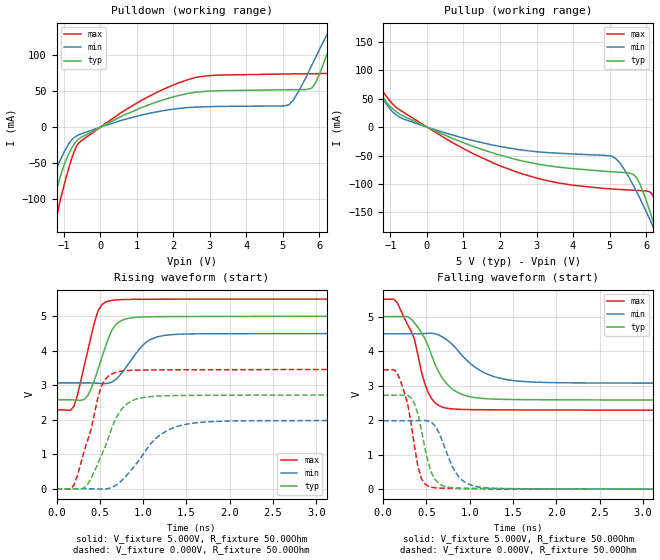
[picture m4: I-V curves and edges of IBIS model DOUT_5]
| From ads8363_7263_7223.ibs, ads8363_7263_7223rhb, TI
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|   Output 5.0V Model
[Model]   DOUT_5
Model_type   Output
|Signals   SDOA, SDOB
Vmeas = 2.413V
Cref = 30.00pF
| C_comp   obtained at 36MHz
| variable   typ   min   max
|C_comp Output Low
C_comp   3.625pF   2.838pF   4.470pF
|C_comp Output High
|C_comp   3.802pF   3.032pF   4.673pF
[Model Spec]
Vmeas   2.41V   2.19V   2.78V
Vref   2.50V   0.50V   3.00V
|Junction Temperature
[Temperature Range]   40.0   125.0   -40.0
[Voltage range]   5.0V   4.50V   5.50V
[pullup reference]   5.0V   4.50V   5.50V
[power clamp reference]   5.0V   4.50V   5.50V
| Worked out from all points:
|   slope of the pulldown table from 0 to 0.75 V, typ, clamps not added: 39.7 ohm
|   slope of the pullup table from 0 to 0.75 V, typ, clamps not added: 35.6 ohm
|   falling waveform, V_fixture 5.000V, R_fixture 50.00Ohm: 20-80 % time 285ps typ, 394ps min, 237ps max; typ from 5 V to 2.58 V
|   rising waveform, V_fixture 5.000V, R_fixture 50.00Ohm: 20-80 % time 201ps typ, 268ps min, 180ps max; typ from 2.58 V to 5 V
|   rising waveform, V_fixture 0.000V, R_fixture 50.00Ohm: 20-80 % time 270ps typ, 399ps min, 217ps max; typ from 0 V to 2.72 V
|   falling waveform, V_fixture 0.000V, R_fixture 50.00Ohm: 20-80 % time 148ps typ, 211ps min, 150ps max; typ from 2.72 V to 0 V
[Pulldown]
|   Voltage   I(typ)   I(min)   I(max)
-5V       -965.9mA   -669mA     -1.352A
-1.794V   -213.8mA   -138mA     -310.7mA
-1.449V   -138.1mA   -89.44mA   -200.4mA
-1.248V   -96.79mA   -63.62mA   -139.3mA
-614.4mV  -17.36mA   -11.32mA   -23.56mA
1.619V    36.23mA    21.99mA    50.12mA
2.89V     49.87mA    28.39mA    71.3mA
5.168V    52.02mA    31.06mA    73.97mA
5.787V    54mA       85.49mA    74.31mA
6.394V    127.3mA    145.7mA    77.14mA
6.895V    190.4mA    185.8mA    160.7mA
9.998V    382.4mA    320.5mA    444.5mA
[Pullup]
|   Voltage   I(typ)   I(min)   I(max)
-5V       320.7mA    274.7mA    381.1mA
-2.705V   207.7mA    175.6mA    249.5mA
-2.326V   179.2mA    150.8mA    217.1mA
-2.002V   149.2mA    125.6mA    181.5mA
-1.115V   44.11mA    40.77mA    54.33mA
0V        -55.47nA   -67.38nA   -44.41nA
2.575V    -59.02mA   -40.11mA   -81.46mA
5.074V    -78.59mA   -51.47mA   -108.9mA
5.721V    -87.38mA   -110.8mA   -111.3mA
6.237V    -174.7mA   -181.8mA   -125.7mA
6.582V    -249.3mA   -234.2mA   -198.1mA
9.998V    -1.057A    -814.1mA   -1.31A
[Ramp]
R_load = 50.00Ohm
|   typ   min   max
dV/dt_r   1.631V/269.984ps   1.188V/398.909ps   2.074V/216.671ps
dV/dt_f   1.452V/284.679ps 858.201mV/394.352ps   1.926V/236.502ps
[Falling Waveform]
V_fixture = 5.000V
V_fixture_min = 4.500V
V_fixture_max = 5.500V
R_fixture = 50.00Ohm
|   Time   V(typ)   V(min)   V(max)
0s        5V         4.5V       5.5V
160ps     5V         4.5V       5.411V
320ps     4.934V     4.499V     4.589V
360ps     4.823V     4.499V     4.351V
520ps     4.151V     4.516V     2.8V
680ps     3.23V      4.416V     2.38V
920ps     2.736V     3.85V      2.309V
1.16ns    2.626V     3.383V     2.3V
1.44ns    2.599V     3.169V     2.296V
4ns       2.58V      3.07V      2.289V
[Rising Waveform]
V_fixture = 5.000V
V_fixture_min = 4.500V
V_fixture_max = 5.500V
R_fixture = 50.00Ohm
|   Time   V(typ)   V(min)   V(max)
0s        2.58V      3.07V      2.289V
200ps     2.576V     3.07V      2.388V
360ps     2.703V     3.069V     3.991V
480ps     3.465V     3.06V      5.164V
600ps     4.366V     3.06V      5.442V
680ps     4.747V     3.161V     5.475V
760ps     4.889V     3.378V     5.486V
1.04ns    4.985V     4.257V     5.494V
1.24ns    4.992V     4.442V     5.496V
4ns       5V         4.5V       5.5V
[Rising Waveform]
V_fixture = 0.000V
V_fixture_min = 0.000V
V_fixture_max = 0.000V
R_fixture = 50.00Ohm
|   Time   V(typ)   V(min)   V(max)
0s        -1.322uV   -2.137uV   -813.2nV
200ps     -2.857mV   233uV      101.3mV
360ps     131.9mV    50.68uV    1.41V
520ps     971.4mV    -8.564mV   2.979V
680ps     2.017V     90.36mV    3.372V
800ps     2.433V     360.2mV    3.424V
920ps     2.598V     720mV      3.438V
1.16ns    2.685V     1.486V     3.446V
1.48ns    2.706V     1.861V     3.45V
4ns       2.718V     1.981V     3.456V
[Falling Waveform]
V_fixture = 0.000V
V_fixture_min = 0.000V
V_fixture_max = 0.000V
R_fixture = 50.00Ohm
|   Time   V(typ)   V(min)   V(max)
0s        2.718V     1.981V     3.456V
160ps     2.719V     1.981V     3.375V
280ps     2.724V     1.981V     2.499V
320ps     2.647V     1.982V     1.955V
400ps     2.184V     1.987V     673.3mV
520ps     771.2mV    1.976V     86.03mV
680ps     109.5mV    1.416V     27.89mV
840ps     33.41mV    470.8mV    21.15mV
1.08ns    20.04mV    73.09mV    14.28mV
4ns       -1.322uV   -2.137uV   -813.2nV
